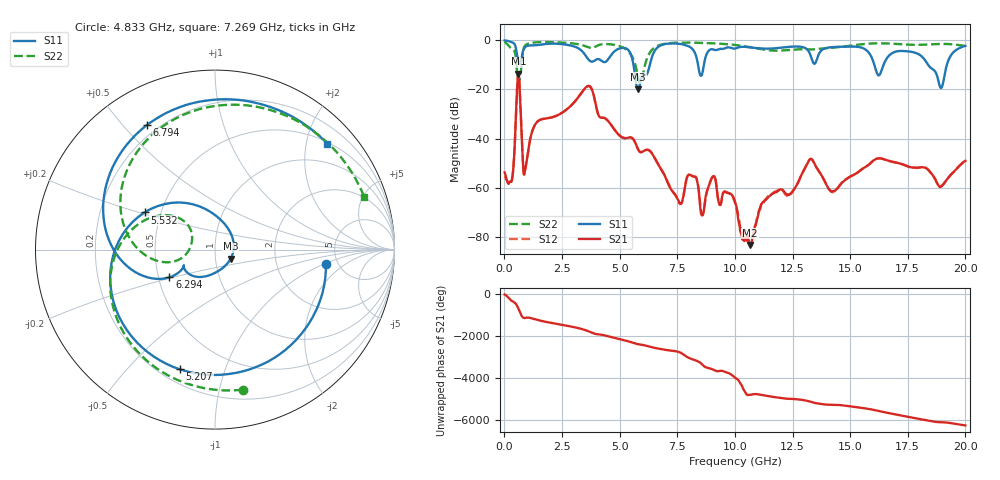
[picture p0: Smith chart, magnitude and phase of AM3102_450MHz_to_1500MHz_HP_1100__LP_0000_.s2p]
!Agilent Technologies,E8364B,MY43040894,A.07.50.67
!Agilent E8364B: A.07.50.67
!Date: Thursday, January 11, 2018 06:31:45
!Correction: S11(Full 2 Port(1,2))
!S21(Full 2 Port(1,2))
!S12(Full 2 Port(1,2))
!S22(Full 2 Port(1,2))
!S2P File: Measurements: S11, S21, S12, S22:
# Hz S  dB  R 50
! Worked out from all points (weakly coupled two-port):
!   1601 points, 10 MHz to 20 GHz, reference 50 ohm
!   highest |S21| = -13.61 dB at 609.7 MHz (marker M1); lowest = -83.2 dB at 10.65 GHz (marker M2)
!   lowest |S11| = -19.9 dB at 5.807 GHz (marker M3), VSWR 1.22, Z = 59.2 - j6.04 ohm
!   |S11| at or under -10 dB: 5.602 GHz to 6.308 GHz (706.6 MHz wide, 11.9 % of centre); 16.05 GHz to 16.45 GHz (400 MHz wide, 2.46 % of centre); 18.38 GHz to 19.2 GHz (810.9 MHz wide, 4.32 % of centre)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
!   |S22| runs from -17.4 to -0.6 dB; largest |S21 - S12| = 0.00078
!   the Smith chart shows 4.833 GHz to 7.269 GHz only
!   S11 on the Smith chart (normalised r, x): 4.833 GHz: 4.00, -1.05; 5.207 GHz: 0.28, -0.71; 5.532 GHz: 0.40, +0.21; 6.294 GHz: 0.57, -0.19; 6.794 GHz: 0.16, +0.58; 7.269 GHz: 0.53, +2.42
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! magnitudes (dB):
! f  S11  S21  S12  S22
! 10 MHz  -0.1  -53.8  -55.4  -0.6
! 322.3 MHz  -0.8  -57.2  -56.6  -3.5
! 609.7 MHz  -8.9  -13.6  -13.6  -16.0
! 897.1 MHz  -2.8  -52.8  -52.9  -2.2
! 1.384 GHz  -2.0  -33.6  -33.6  -0.8
! 3.346 GHz  -4.2  -21.4  -21.4  -1.9
! 4.833 GHz  -4.1  -37.1  -37.1  -2.0
! 5.207 GHz  -3.2  -39.8  -39.8  -3.3
! 5.532 GHz  -7.1  -39.7  -39.7  -6.5
! 5.807 GHz  -19.9  -44.5  -44.5  -15.3
! 6.294 GHz  -10.5  -44.9  -44.9  -5.3
! 6.682 GHz  -2.6  -50.6  -50.7  -2.2
! 6.794 GHz  -2.0  -52.4  -52.4  -1.8
! 7.269 GHz  -1.3  -61.2  -61.0  -1.1
! 8.531 GHz  -14.4  -70.3  -69.3  -1.1
! 10.01 GHz  -3.4  -65.7  -66.0  -1.9
! 10.65 GHz  -2.9  -83.2  -83.2  -2.8
! 13.34 GHz  -7.8  -48.4  -48.5  -3.8
! 14.24 GHz  -2.8  -61.4  -61.8  -3.1
! 16.68 GHz  -6.4  -49.1  -49.1  -1.3
! 18.94 GHz  -19.4  -59.6  -59.3  -1.5
! 20 GHz  -2.3  -49.0  -49.0  -2.3
